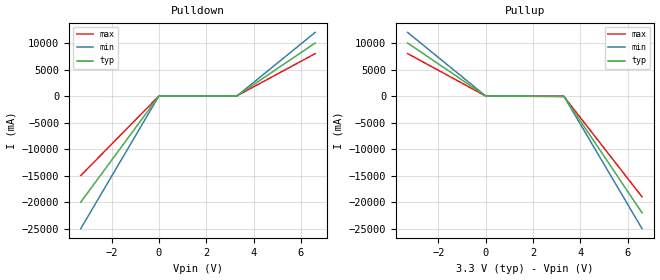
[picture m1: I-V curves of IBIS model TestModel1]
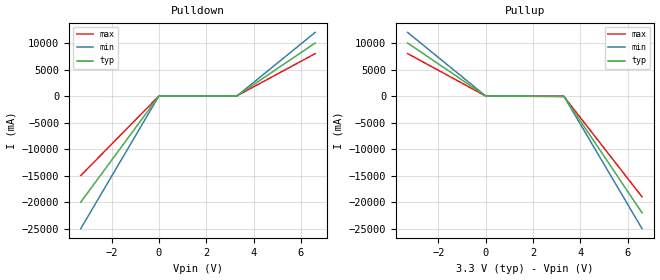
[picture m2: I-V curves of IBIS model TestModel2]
|DESCRIPTION OF BUG:
|Section 9 of the IBIS 3.2 specification, under "Notes on Data Derivation
|Method,"
|describes the proper assignment of values to "min" and "max" data columns:
|   "The 'min' and 'max' columns for all remaining keywords and
|   subparameters will contain the smallest and largest magnitude
|   values.  This applies to the [Model] subparameter C_comp as
|   well..."
|Currently, the parser does not generate any message to the user when the
|numerically-largest C_comp value appears under the "min" data column.
|Similarly, no error is flagged when the numerically-smallest C_comp value
|appears under the "max" data column.  Currently, several vendors' own
|IBIS converters flag this mis-ordering as an error.  As many tool vendors
|allow the user to map any C_comp value to any device corner, independently
|of VT and IV curve data, strict numerical ordering of C_comp should be
|enforced.
|Some indication -- most appropriately, an error -- should be made by the
|parser of the incorrect ordering of C_comp values.
|An example:
|  ERROR (line  xxx) - A model's "min" C_comp must be the smallest
|  value listed while "max" C_comp must be the largest value listed.
|This bug also applies to DOS32 IBISCHK3 v3.2.5.
[IBIS Ver]   3.2
[File Name]   bug50.ibs
[File Rev]   0.0
[Date]   08-November-2000
[Source]   File created from specification
[Disclaimer]
   (C) Copyright 2000 Intel Corp.
   All rights reserved
   This model is for demonstration purposes only.
[Component]   GENERIC_IBIS
[Manufacturer]   Intel Corp.
[Package]
|   typ   min   max
R_pkg   6.0mO   5.0mO   7.0mO
L_pkg   5.0nH   2.0nH   8.0nH
C_pkg   1.0pF   0.5pF   1.5pF
[Pin]   signal_name   model_name   R_pin   L_pin   C_pin
   A1   TestSignal1   TestModel1
   A2   TestSignal2   TestModel2
| Models and submodels in the file (2): TestModel1 (Output), TestModel2 (Output)
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|* this should give a warning for C_Comp
[Model]   TestModel1
Model_type   Output
Polarity   Non-Inverting
Cref = 10.0pF
C_comp   5.00pF   40.00pF   1.00pF
[Temperature Range]   27.00   100.00   0.00
[Voltage Range]   3.30V   3.00V   3.60V
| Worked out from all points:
|   slope of the pulldown table from 0 to 0.495 V, typ, clamps not added: 82.5 ohm
|   slope of the pullup table from 0 to 0.495 V, typ, clamps not added: 50.8 ohm
[Pulldown]
| voltage   I(typ)   I(min)   I(max)
-3.3V     -20A       -25A       -15A
0V        0A         -5nA       5nA
3.3V      40mA       32mA       48mA
6.6V      10A        12A        8A
[Pullup]
| voltage   I(typ)   I(min)   I(max)
-3.3V     10A        12A        8A
0V        0A         -300nA     300nA
3.3V      -65mA      -40mA      -80mA
6.6V      -22A       -25A       -19A
[Ramp]
| variable   typ   min   max
dV/dt_r   0.35/1.6n   0.25/1.8n   0.45/1.5n
dV/dt_f   0.35/1.6n   0.25/1.8n   0.45/1.5n
R_load = 50.000
| * this should not give any warning for C_comp
[Model]   TestModel2
Model_type   Output
Polarity   Non-Inverting
Cref = 10.0pF
C_comp   5.00pF   4.00pF   10.00pF
[Temperature Range]   27.00   100.00   0.00
[Voltage Range]   3.30V   3.00V   3.60V
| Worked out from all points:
|   slope of the pulldown table from 0 to 0.495 V, typ, clamps not added: 82.5 ohm
|   slope of the pullup table from 0 to 0.495 V, typ, clamps not added: 50.8 ohm
[Pulldown]
| voltage   I(typ)   I(min)   I(max)
-3.3V     -20A       -25A       -15A
0V        0A         -5nA       5nA
3.3V      40mA       32mA       48mA
6.6V      10A        12A        8A
[Pullup]
| voltage   I(typ)   I(min)   I(max)
-3.3V     10A        12A        8A
0V        0A         -300nA     300nA
3.3V      -65mA      -40mA      -80mA
6.6V      -22A       -25A       -19A
[Ramp]
| variable   typ   min   max
dV/dt_r   0.35/1.6n   0.25/1.8n   0.45/1.5n
dV/dt_f   0.35/1.6n   0.25/1.8n   0.45/1.5n
R_load = 50.000
